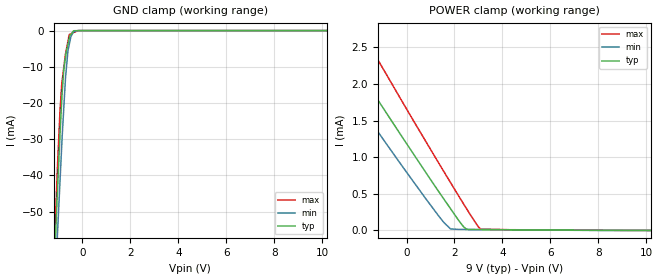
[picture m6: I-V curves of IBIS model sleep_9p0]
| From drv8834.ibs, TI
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|   sleep_9p0 Model
[Model]   sleep_9p0
Model_type   Input
Vinl = 0.7
Vinh = 2
|   typ   min   max
|   (nom PVT)   (fast PVT)   (slow PVT)
|C_comp from frequency sweep method (F=250KHz)
|Average
|C_comp   2.499e-12   2.286e-12   2.718e-12
|C_comp from LC tank measurement(L=1nH)
|Average
|Resonant Frequency(Hz)   4.480e+09   4.560e+09   4.400e+09
 C_comp   1.263e-12   1.219e-12   1.310e-12
| Where nom  PVT is Nominal Process, 9V, 27C
|   Fast PVT is Strong Process,  9.9V, -40C
|   Slow PVT is Weak Process,   8.1V, 125C
[Voltage Range]   9   8.1   9.9
|Ambient Temperature   25   150   -40
|Junction Temperature
[Temperature Range]   27   125   -40
[Power Clamp Reference]   9   8.1   9.9
[GND Clamp Reference]   0   0   0
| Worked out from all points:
|   GND clamp passes 1 mA (typ) near -0.47 V on its own axis
[GND Clamp]
|   Voltage   I(typ)   I(min)   I(max)
-9V       -1.598A    -1.486A    -1.684A
-1.197V   -69.78mA   -80.18mA   -65.58mA
-1.053V   -46.77mA   -58.72mA   -40.68mA
-1.03V    -43.3mA    -55.38mA   -36.76mA
-930.6mV  -28.66mA   -41.72mA   -22.22mA
-861.3mV  -19.75mA   -32.17mA   -15.18mA
-765mV    -10.45mA   -20.54mA   -9.838mA
-696.6mV  -7.113mA   -12.73mA   -6.302mA
-599.4mV  -3.788mA   -5.581mA   -2.968mA
-544.5mV  -2.138mA   -3.838mA   -1.084mA
-360mV    -45.21uA   -327.4uA   -538.2uA
18V       0A         0A         0A
[POWER Clamp]
|   Voltage   I(typ)   I(min)   I(max)
-9V       9.488mA    9.67mA     11.49mA
-3.694V   3.762mA    3.415mA    4.462mA
-2.94V    2.91mA     2.587mA    3.378mA
-2.812V   2.769mA    2.45mA     3.241mA
-2.475V   2.432mA    2.092mA    3.05mA
-2.219V   2.299mA    1.851mA    2.906mA
-2.009V   2.19mA     1.731mA    2.788mA
-1.633V   2.001mA    1.554mA    2.576mA
1.839V    295.6uA    21.57uA    651.6uA
2.493V    18.54uA    13.74uA    302.6uA
3.089V    11.63uA    12.28uA    18.95uA
18V       0A         0A         0A
